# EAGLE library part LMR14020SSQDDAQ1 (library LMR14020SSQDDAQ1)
Automotive 40V, 2A SIMPLE SWITCHER, 2.2MHz Step-Down Regulator with 40uA IQ Source: Datasheet
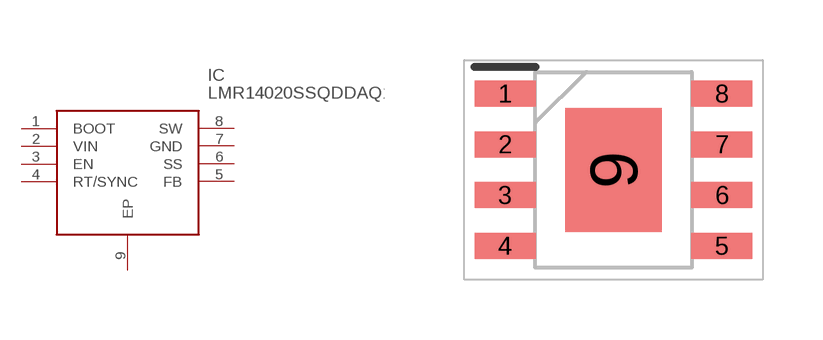
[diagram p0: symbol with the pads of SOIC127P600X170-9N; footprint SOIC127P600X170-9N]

Designator prefix IC

## LMR14020SSQDDAQ1 (Description: Automotive 40V, 2A SIMPLE SWITCHER, 2.2MHz Step-Down Regulator with 40uA IQ; Height: 1.7mm; Manufacturer_Name: Texas Instruments; Manufacturer_Part_Number: LMR14020SSQDDAQ1; Mouser_Part_Number: 595-LMR14020SSQDDAQ1; Mouser_Price-Stock: https://www.mouser.co.uk/ProductDetail/Texas-Instruments/LMR14020SSQDDAQ1?qs=diC8vqfyxkp45LTZX%252BiGRA%3D%3D)  [SOIC127P600X170-9N]
1  BOOT
2  VIN
3  EN
4  RT/SYNC
5  FB
6  SS
7  GND
8  SW
9  EP

## Footprint SOIC127P600X170-9N (pad centres in mm)
DDA (R-PDSO-G8)-ren1
smd 1.525 x 0.65: 1 -2.712,1.905; 2 -2.712,0.635; 3 -2.712,-0.635; 4 -2.712,-1.905; 5 2.712,-1.905; 6 2.712,-0.635; 7 2.712,0.635; 8 2.712,1.905
smd 2.4 x 3.1: 9 0,0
